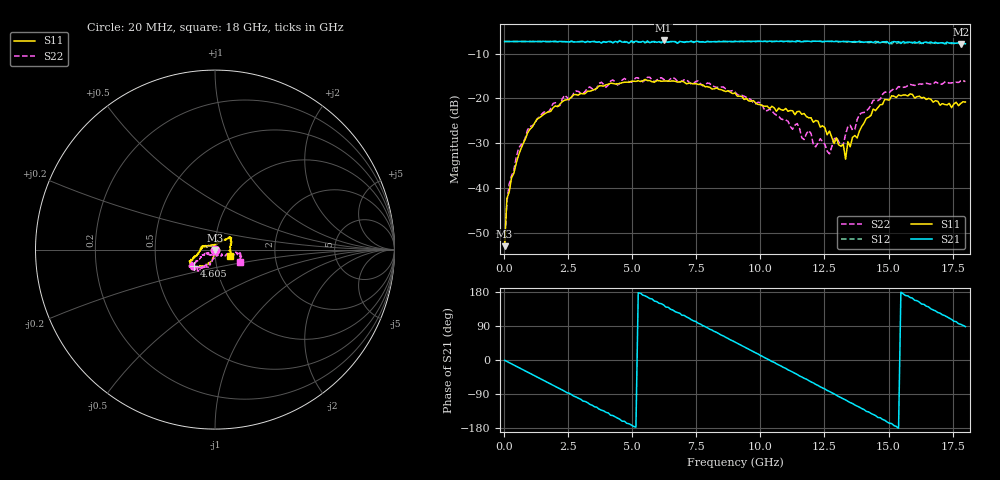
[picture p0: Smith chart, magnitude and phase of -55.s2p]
!Agilent Technologies,N5230A,US43500223,A.07.50.48
!Agilent N5230A: A.07.50.48
!Date: Wednesday, February 17, 2016 13:36:29
!Correction: S11(Full 2 Port(1,2))
!S21(Full 2 Port(1,2))
!S12(Full 2 Port(1,2))
!S22(Full 2 Port(1,2))
!S2P File: Measurements: S11, S21, S12, S22:
# Hz S  RI  R 50
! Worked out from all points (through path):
!   201 points, 20 MHz to 18 GHz, reference 50 ohm
!   highest |S21| = -7.07 dB at 6.223 GHz (marker M1); lowest = -7.9 dB at 17.82 GHz (marker M2)
!   group delay of S21, straight-line fit = 97.5 ps
!   lowest |S11| = -52.9 dB at 20 MHz (marker M3), VSWR 1.00, Z = 50 - j0.222 ohm
!   |S11| at or under -10 dB: start of sweep to end of sweep
!   |S22| runs from -52.2 to -15.3 dB; largest |S21 - S12| = 0.036
!   S11 on the Smith chart (normalised r, x): 20 MHz: 1.00, -0.00; 4.605 GHz: 0.78, -0.15; 18 GHz: 1.18, -0.08
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2e7  -0.000425 -0.00223  0.4309 -0.00555  0.4309 -0.00603  0.00139 -0.00204
1.099e8  0.00324 -0.007  0.4296 -0.0293  0.4304 -0.0282  0.00137 -0.00689
5.594e8  -0.00128 -0.0231  0.4066 -0.1437  0.406 -0.1446  0.000445 -0.0276
9.19e8  -0.00854 -0.0405  0.3661 -0.2286  0.3652 -0.2299  -0.00674 -0.0446
3.0766e9  -0.064 -0.0925  -0.1357 -0.4106  -0.1329 -0.4108  -0.0634 -0.0939
4.6049e9  -0.1179 -0.0926  -0.403 -0.1346  -0.3993 -0.1308  -0.1232 -0.1023
6.0433e9  -0.1404 -0.0716  -0.3709 0.2152  -0.3668 0.2279  -0.1423 -0.0891
6.2231e9  -0.1404 -0.0691  -0.3642 0.252  -0.3493 0.2552  -0.1317 -0.0983
7.5716e9  -0.1309 -0.0586  -0.0526 0.4297  -0.0447 0.4251  -0.1313 -0.0862
9.01e9  -0.1089 -0.0372  0.2936 0.3183  0.3024 0.3087  -0.0996 -0.0637
1.05383e10  -0.0787 0.00313  0.4284 -0.0457  0.4295 -0.0607  -0.0601 -0.0318
1.18868e10  -0.0575 0.0205  0.2534 -0.3523  0.24 -0.3634  -0.0358 -0.0256
1.20666e10  -0.0515 0.017  0.2143 -0.3774  0.2004 -0.3869  -0.0179 -0.0247
1.26959e10  -0.036 0.0242  0.0523 -0.4292  0.0374 -0.4311  -0.00467 -0.0237
1.29656e10  -0.0263 0.0252  -0.0208 -0.4329  -0.0463 -0.4307  0.00672 -0.0366
1.32353e10  -0.0156 0.0265  -0.094 -0.4221  -0.1126 -0.4152  0.0114 -0.0285
1.33252e10  -0.00442 0.0206  -0.1135 -0.4165  -0.1315 -0.4057  0.0177 -0.0358
1.34151e10  -0.00285 0.033  -0.141 -0.4088  -0.1542 -0.3974  0.0309 -0.0379
1.50333e10  0.0721 0.0633  -0.3958 -0.0922  -0.4095 -0.0732  0.1161 -0.0143
1.6202e10  0.0886 0.0584  -0.384 0.1965  -0.3514 0.2097  0.1427 -0.0267
1.78202e10  0.0841 -0.0265  -0.029 0.4026  -0.0007 0.403  0.1464 -0.0566
1.8e10  0.0851 -0.0331  0.0133 0.4073  0.0429 0.4038  0.1378 -0.0689
